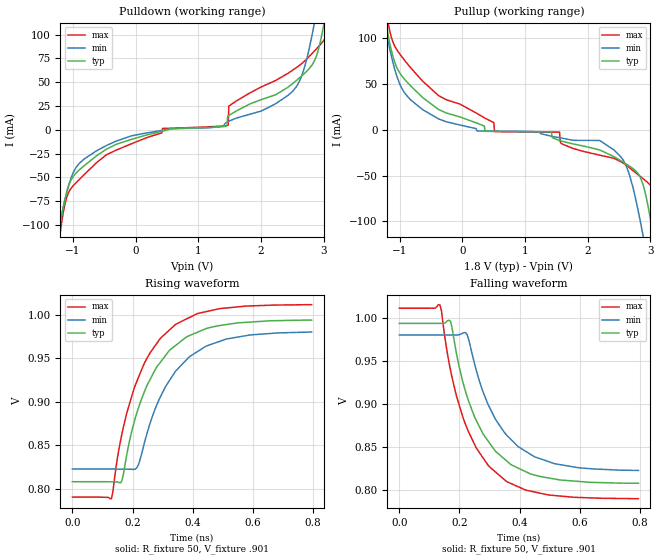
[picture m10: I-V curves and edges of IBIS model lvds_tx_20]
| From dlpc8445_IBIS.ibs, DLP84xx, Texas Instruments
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|   MODEL lvds_tx_20
[Model] lvds_tx_20
Model_type Output
C_comp 1.366p 914.839f 1.417p
Vmeas = 1.2
Vref = 1.2V
Rref = 50
Cref = 0.5pF
[Model Spec]
[Temperature Range]  40 150 -40
[Voltage Range] 1.8 1.62 1.98
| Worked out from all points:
|   slope of the pulldown table from 0 to 0.27 V, typ, clamps not added: 56 ohm
|   slope of the pullup table from 0 to 0.27 V, typ, clamps not added: 39.4 ohm
|   rising waveform, R_fixture 50, V_fixture .901: 20-80 % time 133ps typ, 140ps min, 132ps max; typ from 0.808 V to 0.994 V
|   falling waveform, R_fixture 50, V_fixture .901: 20-80 % time 129ps typ, 135ps min, 129ps max; typ from 0.994 V to 0.808 V
[Pulldown]
-1.717V   -348.6mA   -301.8mA   -413.4mA
-1.247V   -117.5mA   -111.3mA   -129.3mA
-992.7mV  -48.57mA   -44.45mA   -58.38mA
-622.4mV  -27.19mA   -21.94mA   -34.34mA
430.2mV   -1.356mA   -478.1uA   1.461mA
1.467V    12.83mA    8.326mA    4.628mA
1.488V    15.1mA     9.02mA     24.97mA
2.006V    31.75mA    19.8mA     45.09mA
2.562V    51.55mA    44.91mA    65.13mA
2.837V    70.25mA    106.2mA    81.53mA
3.017V    115.6mA    173.6mA    94.97mA
3.514V    352.8mA    380.6mA    307.6mA
[Pullup]
-1.714V   352.6mA    305.1mA    417.4mA
-1.243V   125.2mA    115.7mA    141.2mA
-989.2mV  60.98mA    48.23mA    81.81mA
-634.8mV  35.28mA    22.04mA    53.13mA
513mV     -1.706mA   -1.514mA   -1.942mA
1.55V     -11.77mA   -8.612mA   -2.533mA
2.19V     -21.97mA   -11.61mA   -27.67mA
2.602V    -36.9mA    -37.86mA   -38.18mA
2.877V    -58.96mA   -114mA     -53.14mA
3.047V    -116.9mA   -179.8mA   -64.92mA
3.205V    -190.8mA   -245.6mA   -118.1mA
3.517V    -348.5mA   -377.8mA   -301mA
[Ramp]
dV/dt_r .112/133.657p .095/140.73p .133/131.887p
dV/dt_f .112/129.415p .095/136.746p .133/128.896p
[Rising Waveform]
R_fixture = 50
V_fixture = .901
V_fixture_min = .901
V_fixture_max = .901
0s        807.9mV    822.4mV    790.1mV
130ps     807.7mV    822.4mV    788.4mV
165ps     809.4mV    822.3mV    863.5mV
205ps     875.9mV    822mV      915mV
220ps     893.2mV    828mV      928.1mV
275ps     936.5mV    891.5mV    964.2mV
340ps     963.6mV    933.4mV    987.7mV
390ps     975.9mV    951.7mV    996.7mV
510ps     988.4mV    971.6mV    1.007V
795ps     993.6mV    979.9mV    1.011V
[Falling Waveform]
R_fixture = 50
V_fixture = .901
V_fixture_min = .901
V_fixture_max = .901
0s        993.8mV    980.3mV    1.011V
135ps     993.9mV    980.3mV    1.015V
170ps     996.4mV    980.3mV    939.9mV
215ps     921.1mV    983mV      881.3mV
230ps     904.1mV    976mV      868mV
280ps     864.6mV    913mV      836.9mV
355ps     834.8mV    864.7mV    810.7mV
445ps     818.2mV    839.9mV    798.4mV
515ps     813.2mV    831.1mV    794mV
795ps     808.2mV    823.1mV    790.3mV
